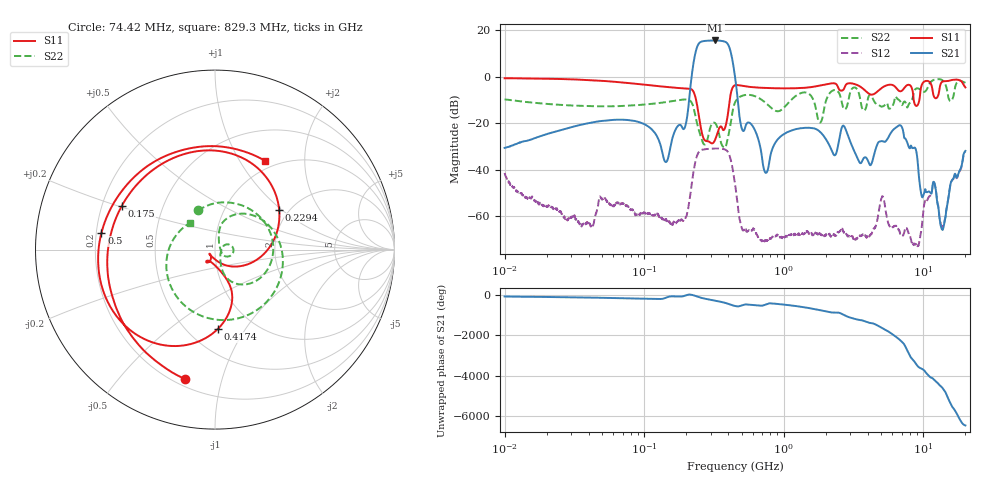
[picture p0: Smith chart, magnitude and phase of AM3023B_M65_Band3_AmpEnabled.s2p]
!Agilent Technologies,E8364B,MY43040894,A.07.50.67
!Agilent E8364B: A.07.50.67
!Date: Tuesday, October 27, 2020 10:52:46
!Correction: S11(Full 2 Port(1,2))
!S21(Full 2 Port(1,2))
!S12(Full 2 Port(1,2))
!S22(Full 2 Port(1,2))
!S2P File: Measurements: S11, S21, S12, S22:Log Frequency Sweep
# Hz S  dB  R 50
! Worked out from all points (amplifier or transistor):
!   3201 points, 10 MHz to 20 GHz, reference 50 ohm
!   highest |S21| = 15.6 dB at 323.8 MHz (marker M1)
!   |S21| within 3 dB of that: 238.7 MHz to 407.5 MHz (168.9 MHz wide, 52.3 % of centre)
!   unconditionally stable (mu >= 1): start of sweep to end of sweep
!   at 35.47 MHz: K = 2094.54, MAG = -14.4 dB, |S12| = -64.3 dB
!   at 447.2 MHz: K = 52.30, MAG = 2.9 dB, |S12| = -46.1 dB
!   at 20 GHz: K = 238.63, MAG = -26.5 dB, |S12| = -32.4 dB
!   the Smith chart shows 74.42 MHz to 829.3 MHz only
!   S11 on the Smith chart (normalised r, x): 74.42 MHz: 0.24, -0.77; 175 MHz: 0.28, +0.21; 229.4 MHz: 1.78, +0.96; 417.4 MHz: 0.69, -0.76; 500 MHz: 0.22, +0.07; 829.3 MHz: 0.88, +1.29
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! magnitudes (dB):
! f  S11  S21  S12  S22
! 10 MHz  -0.7  -30.6  -41.4  -9.7
! 35.55 MHz  -1.3  -20.6  -64.2  -12.5
! 74.42 MHz  -2.6  -18.5  -55.6  -12.5
! 126.1 MHz  -4.0  -26.7  -59.4  -11.3
! 144 MHz  -4.4  -36.6  -61.5  -10.9
! 175 MHz  -4.8  -21.0  -61.9  -10.1
! 198.5 MHz  -5.0  -20.5  -60.4  -9.8
! 229.4 MHz  -7.5  8.5  -38.4  -15.1
! 323.8 MHz  -26.8  15.6  -30.9  -20.1
! 417.4 MHz  -7.1  10.4  -35.8  -19.7
! 447.2 MHz  -3.6  0.1  -46.1  -11.1
! 500 MHz  -3.9  -22.2  -65.0  -8.3
! 740 MHz  -4.8  -41.3  -70.3  -11.2
! 829.3 MHz  -4.9  -30.9  -68.8  -13.8
! 1.59 GHz  -4.4  -22.0  -67.6  -8.7
! 4.151 GHz  -7.5  -38.0  -68.1  -7.8
! 5.067 GHz  -4.7  -27.7  -51.4  -12.8
! 5.639 GHz  -3.5  -25.9  -63.3  -13.6
! 9.047 GHz  -12.3  -35.0  -72.7  -5.0
! 11.92 GHz  -8.5  -45.3  -45.4  -1.3
! 13.64 GHz  -2.1  -65.7  -64.5  -1.4
! 20 GHz  -4.6  -31.9  -32.4  -2.6
